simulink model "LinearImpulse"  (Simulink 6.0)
settings: Solver=ode45  SolverMode=SingleTasking  StartTime=0.0  StopTime=5.0  RelTol=1e-3  AbsTol=1e-6

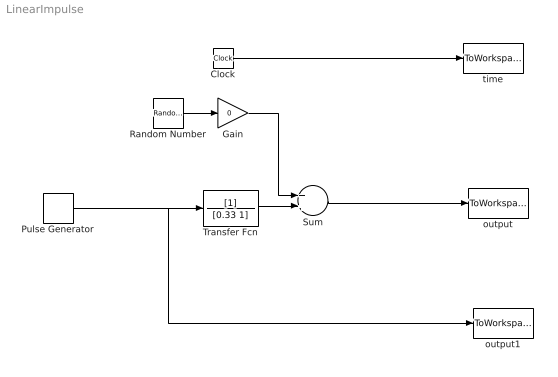
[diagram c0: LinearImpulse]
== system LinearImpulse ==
  Clock : Clock
  Gain : Gain  Gain=0
  Pulse Generator : DiscretePulseGenerator  PulseType=Time based  Period=10  PulseWidth=0.1
  Random Number : RandomNumber  Variance=0.001  SampleTime=0
  Sum : Sum
  Transfer Fcn : TransferFcn  Denominator=[0.33 1]
  output : ToWorkspace  VariableName=y  SampleTime=0.01  SaveFormat=Array
  output1 : ToWorkspace  VariableName=u  SampleTime=0.01  SaveFormat=Array
  time : ToWorkspace  VariableName=t  SampleTime=0.01  SaveFormat=Array
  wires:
  Transfer Fcn/1 -> Sum/2
  Pulse Generator/1 -> Transfer Fcn/1, output1/1
  Clock/1 -> time/1
  Sum/1 -> output/1
  Random Number/1 -> Gain/1
  Gain/1 -> Sum/1
